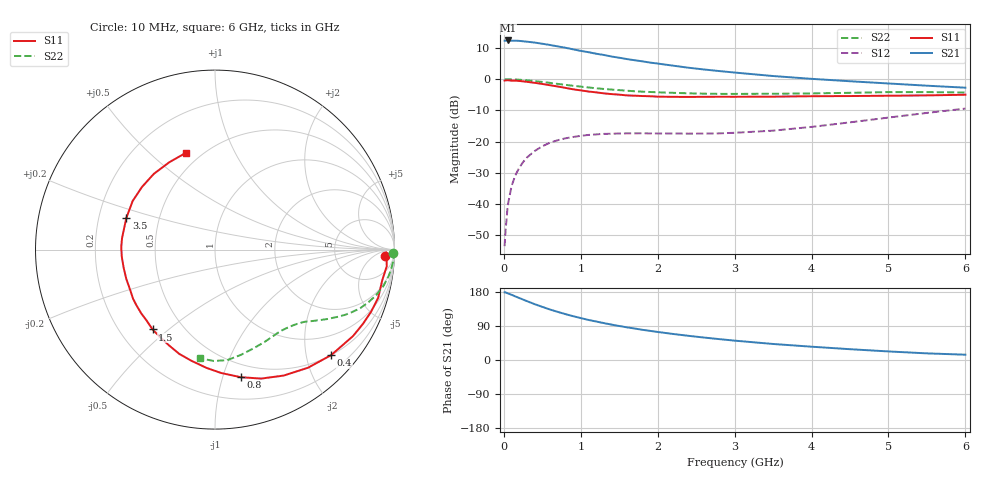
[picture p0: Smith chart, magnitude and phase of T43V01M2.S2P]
! Infineon Technologies  Discrete & RF Semiconductors
! BFR182T
! Si NPN RF Bipolar Junction Transistor in SC75
! VCE = 3 V  IC = 1.2 mA
! Common Emitter S-Parameters:  October  1999
# GHz  S  MA  R  50
!  f  S11  S21  S12  S22
! GHz  MAG  ANG  MAG  ANG  MAG  ANG  MAG  ANG
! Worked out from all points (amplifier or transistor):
!   36 points, 10 MHz to 6 GHz, reference 50 ohm
!   highest |S21| = 12.4 dB at 50 MHz (marker M1)
!   |S21| within 3 dB of that: start of sweep to 932.1 MHz
!   unconditionally stable (mu >= 1): 2.294 GHz to 4.506 GHz
!   at 250 MHz: K = 0.10, MSG = 19.4 dB, |S12| = -26.6 dB
!   at 1.4 GHz: K = 0.63, MSG = 12.4 dB, |S12| = -17.5 dB
!   at 6 GHz: K = 0.83, MSG = 3.4 dB, |S12| = -9.4 dB
!   S11 on the Smith chart (normalised r, x): 10 MHz: 25, -18; 400 MHz: 0.50, -2.50; 800 MHz: 0.38, -1.15; 1.5 GHz: 0.34, -0.44; 3.5 GHz: 0.32, +0.16; 6 GHz: 0.42, +0.66
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0.01  0.9478 -2.2  4.146 178.6  0.0021 87.0  0.9919 -1.2
0.02  0.9548 -0.9  4.142 178.7  0.0034 97.2  0.9929 -0.9
0.05  0.9615 -5.5  4.175 175.9  0.0093 92.9  0.9959 -2.2
0.1  0.9473 -10.4  4.143 172.2  0.0193 85.5  0.9933 -4.3
0.15  0.948 -16.4  4.14 167.7  0.0287 80.4  0.9867 -6.4
0.25  0.9226 -26.6  4.049 159.5  0.0468 74.6  0.969 -10.4
0.4  0.8742 -42.3  3.864 147.4  0.0705 66.1  0.9314 -16.0
0.5  0.8376 -51.8  3.699 140.2  0.084 60.8  0.9024 -19.1
0.6  0.7994 -61.4  3.533 133.2  0.0958 56.4  0.8722 -22.0
0.7  0.7633 -70.3  3.354 127.0  0.1049 52.4  0.8406 -24.4
0.8  0.7252 -78.6  3.19 121.1  0.1127 48.7  0.8114 -26.6
0.9  0.6882 -87.2  3.011 115.6  0.1182 45.5  0.7829 -28.5
1.1  0.6334 -101.9  2.707 105.7  0.1276 40.4  0.736 -31.7
1.3  0.5923 -115.6  2.444 97.4  0.1326 36.7  0.6964 -34.4
1.5  0.5648 -128.0  2.207 89.7  0.1344 34.5  0.6672 -36.7
1.8  0.5365 -144.7  1.932 79.7  0.1357 32.6  0.6304 -40.2
2.2  0.5205 -161.7  1.646 68.7  0.1346 33.3  0.604 -44.6
2.8  0.5225 178.5  1.349 55.1  0.1352 38.7  0.5815 -52.5
3.5  0.5246 160.3  1.123 42.3  0.1494 48.7  0.5838 -61.7
4.5  0.5361 139.4  0.926 28.5  0.203 58.5  0.6042 -76.3
5.5  0.5494 117.5  0.786 17.5  0.2878 59.1  0.6203 -90.9
6  0.5626 106.9  0.73 14.0  0.3373 56.4  0.6108 -97.8
